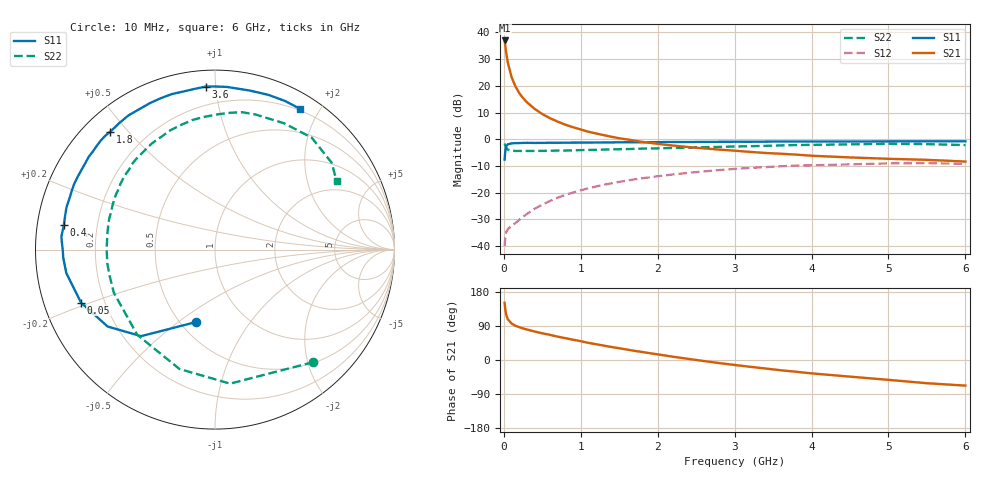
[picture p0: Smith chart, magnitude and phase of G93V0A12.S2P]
! SIEMENS Small Signal Semiconductors
! BFG235
! Si NPN RF Bipolar Junction Transistor in SOT223
! VCE = 3 V  IC = 120 mA
! Common Emitter S-Parameters:  July  1994
# GHz  S  MA  R  50
!  f  S11  S21  S12  S22
! GHz  MAG  ANG  MAG  ANG  MAG  ANG  MAG  ANG
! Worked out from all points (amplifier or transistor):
!   40 points, 10 MHz to 6 GHz, reference 50 ohm
!   highest |S21| = 37.0 dB at 10 MHz (marker M1)
!   |S21| within 3 dB of that: start of sweep to 23.33 MHz
!   unconditionally stable (mu >= 1): 456.6 MHz to 1.522 GHz
!   at 200 MHz: K = 0.80, MSG = 23.7 dB, |S12| = -30.1 dB
!   at 1.5 GHz: K = 1.00, MAG = 7.8 dB, |S12| = -16.0 dB
!   at 6 GHz: K = 0.91, MSG = 0.4 dB, |S12| = -9.2 dB
!   S11 on the Smith chart (normalised r, x): 10 MHz: 0.60, -0.58; 50 MHz: 0.11, -0.19; 400 MHz: 0.08, +0.08; 1.8 GHz: 0.08, +0.45; 3.6 GHz: 0.09, +0.94; 6 GHz: 0.18, +1.76
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0.01  0.4161 -104.4  70.51 151.1  0.01 61.8  0.8321 -48.9
0.02  0.6342 -130.5  54.34 131.7  0.0156 46.3  0.7515 -83.6
0.03  0.7361 -144.4  42.11 120.1  0.0183 39.6  0.6939 -106.6
0.05  0.8028 -158.4  27.77 107.9  0.0206 32.8  0.6426 -132.4
0.1  0.8387 -171.0  14.58 96.3  0.0239 35.9  0.6128 -156.9
0.15  0.8465 -176.8  9.79 90.4  0.027 42.3  0.6049 -167.0
0.2  0.8484 -179.9  7.321 86.6  0.0311 46.6  0.6048 -172.7
0.25  0.8541 177.3  5.898 83.2  0.0355 50.1  0.6029 -176.7
0.3  0.8588 175.1  4.926 80.5  0.04 53.0  0.6039 179.9
0.4  0.8532 170.8  3.708 75.2  0.05 56.0  0.6036 174.9
0.5  0.8563 167.1  2.962 70.4  0.0599 57.1  0.6069 170.8
0.7  0.8595 160.5  2.137 61.6  0.0807 56.7  0.6142 163.5
0.9  0.8657 154.9  1.679 53.5  0.1008 54.0  0.6207 157.2
1.1  0.8667 148.7  1.383 45.2  0.1211 50.7  0.6313 151.0
1.4  0.8727 141.4  1.111 34.3  0.1497 44.6  0.6465 142.5
1.8  0.8792 131.7  0.892 21.1  0.1863 36.0  0.6685 131.5
2.2  0.8897 122.8  0.762 8.6  0.2196 27.0  0.6881 120.7
3.2  0.8982 101.4  0.581 -17.9  0.2903 3.9  0.7415 94.8
3.6  0.9097 93.3  0.536 -27.1  0.3119 -6.1  0.7668 83.8
4.5  0.9071 77.6  0.457 -43.9  0.339 -25.6  0.8021 61.4
5.5  0.9155 64.7  0.412 -61.3  0.3569 -47.2  0.8105 36.7
6  0.9163 58.8  0.383 -67.6  0.3467 -55.4  0.778 29.5
